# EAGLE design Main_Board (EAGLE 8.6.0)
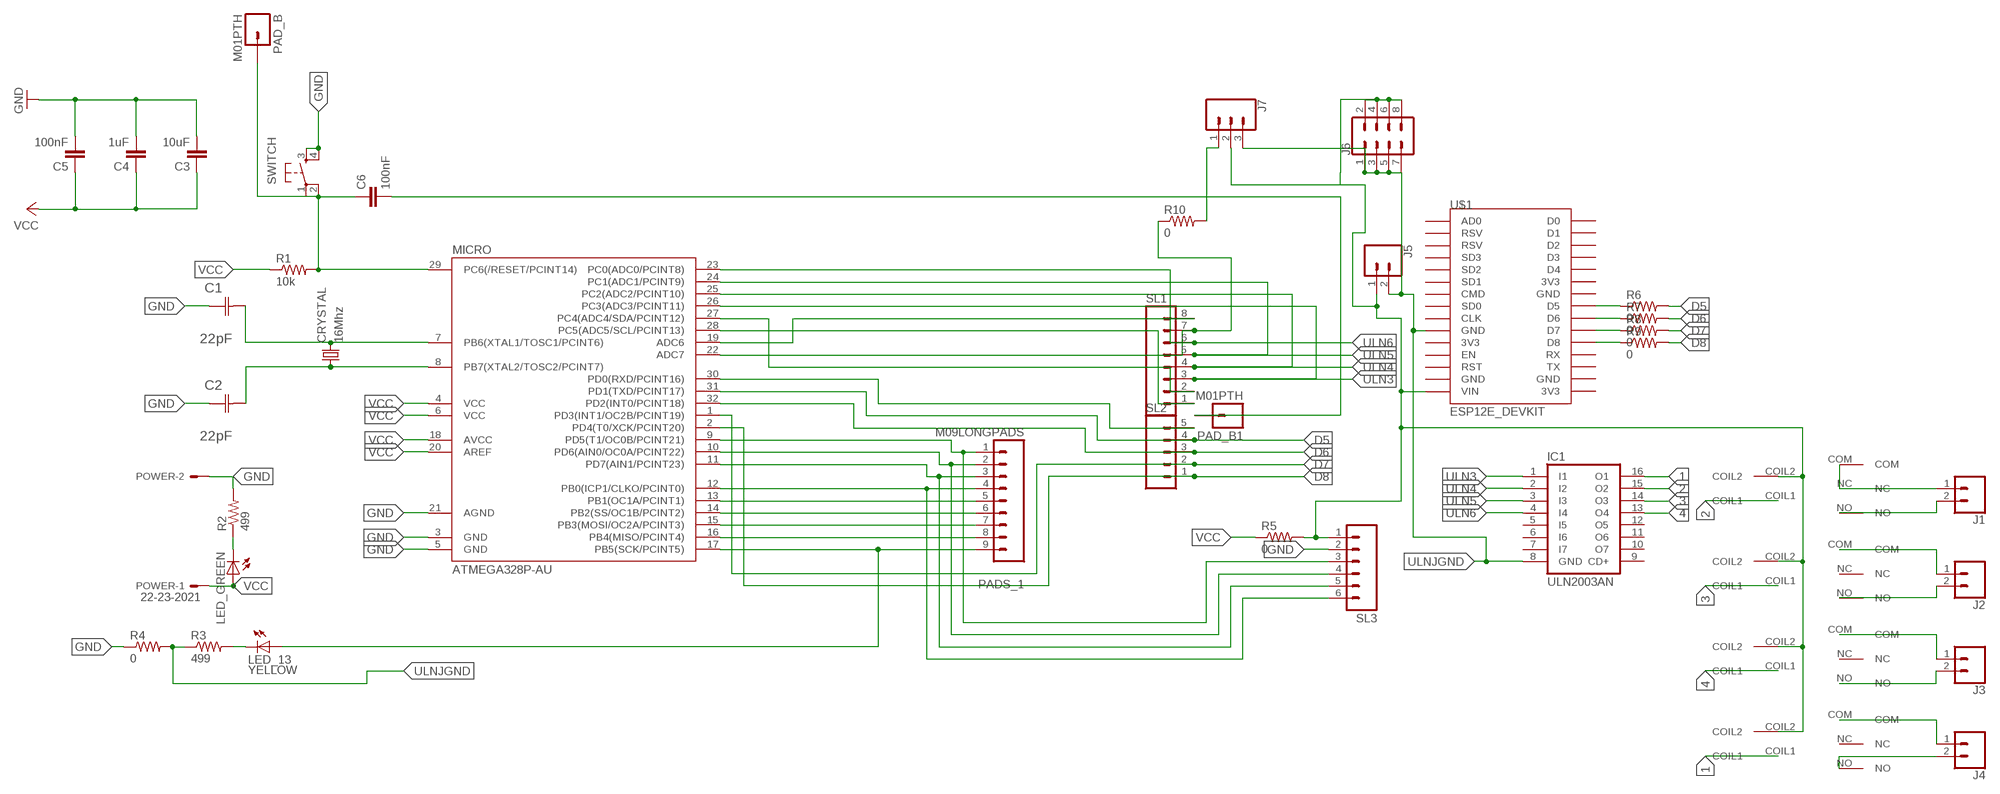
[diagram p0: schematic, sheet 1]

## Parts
C1  22pF  0612ZC225MAT2A  [CAPC3216X178N]
C2  22pF  0612ZC225MAT2A  [CAPC3216X178N]
C3  10uF  CAP1206  [1206]
C4  1uF  CAP1206  [1206]
C5  100nF  CAP1206  [1206]
C6  100nF  CAP1206  [1206]
CRYSTAL  16Mhz  CSM-7X-DU  [CSM-7X-DU]
IC1  ULN2003AN  [DIL16]
J1  CONN_025MM  [SCREWTERMINAL-5MM-2]
J2  CONN_025MM  [SCREWTERMINAL-5MM-2]
J3  CONN_025MM  [SCREWTERMINAL-5MM-2]
J4  CONN_025MM  [SCREWTERMINAL-5MM-2]
J5  CONN_025MM  [SCREWTERMINAL-5MM-2]
J6  CONN_04X2  [2X4]
J7  CONN_03  [1X03]
LED_13  YELLOW  LED1206  [1206]
LED_GREEN  LED1206  [1206]
MICRO  ATMEGA328P-AU  ATMEGA48/88/168-AU  [TQFP32-08]
PAD_B  M01PTH  [1X01]
PAD_B1  M01PTH  [1X01]
PADS_1  M09LONGPADS  [1X09_LONGPADS]
POWER  22-23-2021  [22-23-2021]
R1  10k  RESISTOR1206  [1206]
R2  499  RESISTOR1206  [1206]
R3  499  RESISTOR1206  [1206]
R4  0  RESISTOR1206  [1206]
R5  0  RESISTOR1206  [1206]
R6  0  RESISTOR1206  [1206]
R7  0  RESISTOR1206  [1206]
R8  0  RESISTOR1206  [1206]
R9  0  RESISTOR1206  [1206]
R10  0  RESISTOR1206  [1206]
SL1  M08  [08P]
SL2  M05  [05P]
SL3  M06  [06P]
SWITCH  6MM_SWITCH6MM_SWITCH  [6MM_SWITCH]
U$1  ESP12E_DEVKIT  [ESP12E_DEVKIT]
U$2  1234  [SC05]
U$3  1234  [SC05]
U$4  1234  [SC05]
U$5  1234  [SC05]

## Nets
1: IC1.16(O1) U$5.COIL1
2: IC1.15(O2) U$2.COIL1
3: IC1.14(O3) U$3.COIL1
4: IC1.13(O4) U$4.COIL1
D5: MICRO.31(PD1(TXD/PCINT17)) R6.2 SL2.4
D6: MICRO.32(PD2(INT0/PCINT18)) R7.2 SL2.3
D7: MICRO.1(PD3(INT1/OC2B/PCINT19)) R8.2 SL2.2
D8: MICRO.2(PD4(T0/XCK/PCINT20)) R9.2 SL2.1
GND: C1.1(C1) C2.1(C1) C3.2 C4.2 C5.2 MICRO.3(GND) MICRO.5(GND) MICRO.21(AGND) POWER.2 R2.2 R4.1 SL3.2 SWITCH.3(S) SWITCH.4(S1)
N$1: MICRO.9(PD5(T1/OC0B/PCINT21)) PADS_1.1 SL3.3
N$2: C1.2(C2) CRYSTAL.2 MICRO.7(PB6(XTAL1/TOSC1/PCINT6))
N$3: C6.2 PAD_B1.1
N$4: MICRO.10(PD6(AIN0/OC0A/PCINT22)) PADS_1.2 SL3.4
N$5: MICRO.11(PD7(AIN1/PCINT23)) PADS_1.3 SL3.5
N$6: MICRO.12(PB0(ICP1/CLKO/PCINT0)) PADS_1.4 SL3.6
N$7: MICRO.13(PB1(OC1A/PCINT1)) PADS_1.5
N$8: MICRO.14(PB2(SS/OC1B/PCINT2)) PADS_1.6
N$9: C2.2(C2) CRYSTAL.1 MICRO.8(PB7(XTAL2/TOSC2/PCINT7))
N$10: MICRO.15(PB3(MOSI/OC2A/PCINT3)) PADS_1.7
N$11: MICRO.16(PB4(MISO/PCINT4)) PADS_1.8
N$12: LED_13.1(A) MICRO.17(PB5(SCK/PCINT5)) PADS_1.9
N$13: MICRO.19(ADC6) SL1.8
N$14: MICRO.22(ADC7) R10.1 SL1.7
N$15: J4.2 U$5.NO
N$16: J4.1 U$5.COM
N$17: J7.1 R10.2
N$18: J3.1 U$4.COM
N$19: J3.2 U$4.NO
N$20: MICRO.30(PD0(RXD/PCINT16)) SL2.5
N$21: J2.1 U$3.COM
N$22: J2.2 U$3.NO
N$23: J1.1 U$2.COM
N$24: J1.2 U$2.NO
N$25: J5.1 J6.2 J6.4 J6.6 J6.8 J7.2 R5.2 SL3.1 U$1.VIN U$2.COIL2 U$3.COIL2 U$4.COIL2 U$5.COIL2
N$26: LED_GREEN.2(C) R2.1
N$27: LED_13.2(C) R3.2
N$28: C6.1 MICRO.29(PC6(/RESET/PCINT14)) PAD_B.1 R1.2 SWITCH.1(P) SWITCH.2(P1)
N$31: R9.1 U$1.D8
N$32: R8.1 U$1.D7
N$33: R7.1 U$1.D6
N$34: R6.1 U$1.D5
ULN1: MICRO.28(PC5(ADC5/SCL/PCINT13)) SL1.1
ULN2: MICRO.27(PC4(ADC4/SDA/PCINT12)) SL1.2
ULN3: IC1.1(I1) MICRO.26(PC3(ADC3/PCINT11)) SL1.3
ULN4: IC1.2(I2) MICRO.25(PC2(ADC2/PCINT10)) SL1.4
ULN5: IC1.3(I3) MICRO.24(PC1(ADC1/PCINT9)) SL1.5
ULN6: IC1.4(I4) MICRO.23(PC0(ADC0/PCINT8)) SL1.6
ULNJGND: IC1.8(GND) J5.2 J6.1 J6.3 J6.5 J6.7 J7.3 R3.1 R4.2 U$1.GND@0(GND)
VCC: C3.1 C4.1 C5.1 LED_GREEN.1(A) MICRO.4(VCC) MICRO.6(VCC) MICRO.18(AVCC) MICRO.20(AREF) POWER.1 R1.1 R5.1
Unconnected: IC1.5(I5) IC1.6(I6) IC1.7(I7) IC1.9(CD+) IC1.10(O7) IC1.11(O6) IC1.12(O5) U$1.3V3@0(3V3) U$1.3V3@1(3V3) U$1.3V3@2(3V3) U$1.AD0 U$1.CLK U$1.CMD U$1.D0 U$1.D1 U$1.D2 U$1.D3 U$1.D4 U$1.EN U$1.GND@1(GND) U$1.GND@2(GND) U$1.GND@3(GND) U$1.RST U$1.RSV@0(RSV) U$1.RSV@1(RSV) U$1.RX U$1.SD0 U$1.SD1 U$1.SD2 U$1.SD3 U$1.TX U$2.NC U$3.NC U$4.NC U$5.NC

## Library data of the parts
C1 C2 = AVX_By_element14_Batch_1:0612ZC225MAT2A: Capacitor 1206; MPN: 0612ZC225MAT2A; OC_FARNELL: -; OC_NEWARK: 12N3209; SUPPLIER: AVX; TOLERANCE: ±20%; VALUE: 2.2µF; VOLTAGERATING: 10V
C3-C6 = 01_SparkFun:CAP: Capacitor
CRYSTAL = 01_FAB_Hello:CSM-7X-DU: SMD CRYSTAL; OC_FARNELL: unknown; OC_NEWARK: unknown
IC1 = uln-udn:ULN2003A: DRIVER ARRAY
J1-J5 = SparkFun-Connectors:CONN_02: Multi connection point. Often used as Generic Header-pin footprint for 0.1 inch spaced/style header connections; SF_SKU: PRT-08432
J6 = SparkFun-Connectors:CONN_04X2: Multi connection point. Often used as Generic Header-pin footprint for 0.1 inch spaced/style header connections On any of the 0.1 inch spaced packages, you can populate with these: Break Away Headers - Straight (PRT-00116) Break Away Male Headers - Right Angle (PRT-00553) Female Headers (PRT-00115)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
J7 = SparkFun-Connectors:CONN_03: Multi connection point. Often used as Generic Header-pin footprint for 0.1 inch spaced/style header connections On any of the 0.1 inch spaced packages, you can populate with these: Break Away Headers - Straight (PRT-00116) Break Away Male Headers - Right Angle (PRT-00553) Female Headers (PRT-00115)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
LED_13 LED_GREEN = 01_FAB_Hello:LED
MICRO = atmega8:ATMEGA48/88/168
PAD_B PAD_B1 = 01_SparkFun:M01: Header 1
PADS_1 = 01_SparkFun:M09: Header 9 Standard 9-pin 0.1" header. Use with straight break away headers (SKU : PRT-00116), right angle break away headers (PRT-00553), swiss pins (PRT-00743), machine pins (PRT-00117), and female headers (PRT-00115).
POWER = con-molex:22-23-2021: .100" (2.54mm) Center Header - 2 Pin; MF: MOLEX; MPN: 22-23-2021; OC_FARNELL: 1462926; OC_NEWARK: 25C3832
R1-R10 = 01_SparkFun:RESISTOR: Resistor
SL1 = con-amp-quick:M08: AMP QUICK CONNECTOR; OC_FARNELL: unknown; OC_NEWARK: unknown
SL2 = con-amp-quick:M05: AMP QUICK CONNECTOR; OC_FARNELL: unknown; OC_NEWARK: unknown
SL3 = con-amp-quick:M06: AMP QUICK CONNECTOR; OC_FARNELL: unknown; OC_NEWARK: unknown
SWITCH = 01_FAB_Hello:6MM_SWITCH: OMRON SWITCH
U$1 = nodemcu:ESP12E_DEVKIT: ESP12E DEVKIT BOARD
U$2-U$5 = realySC05:1234

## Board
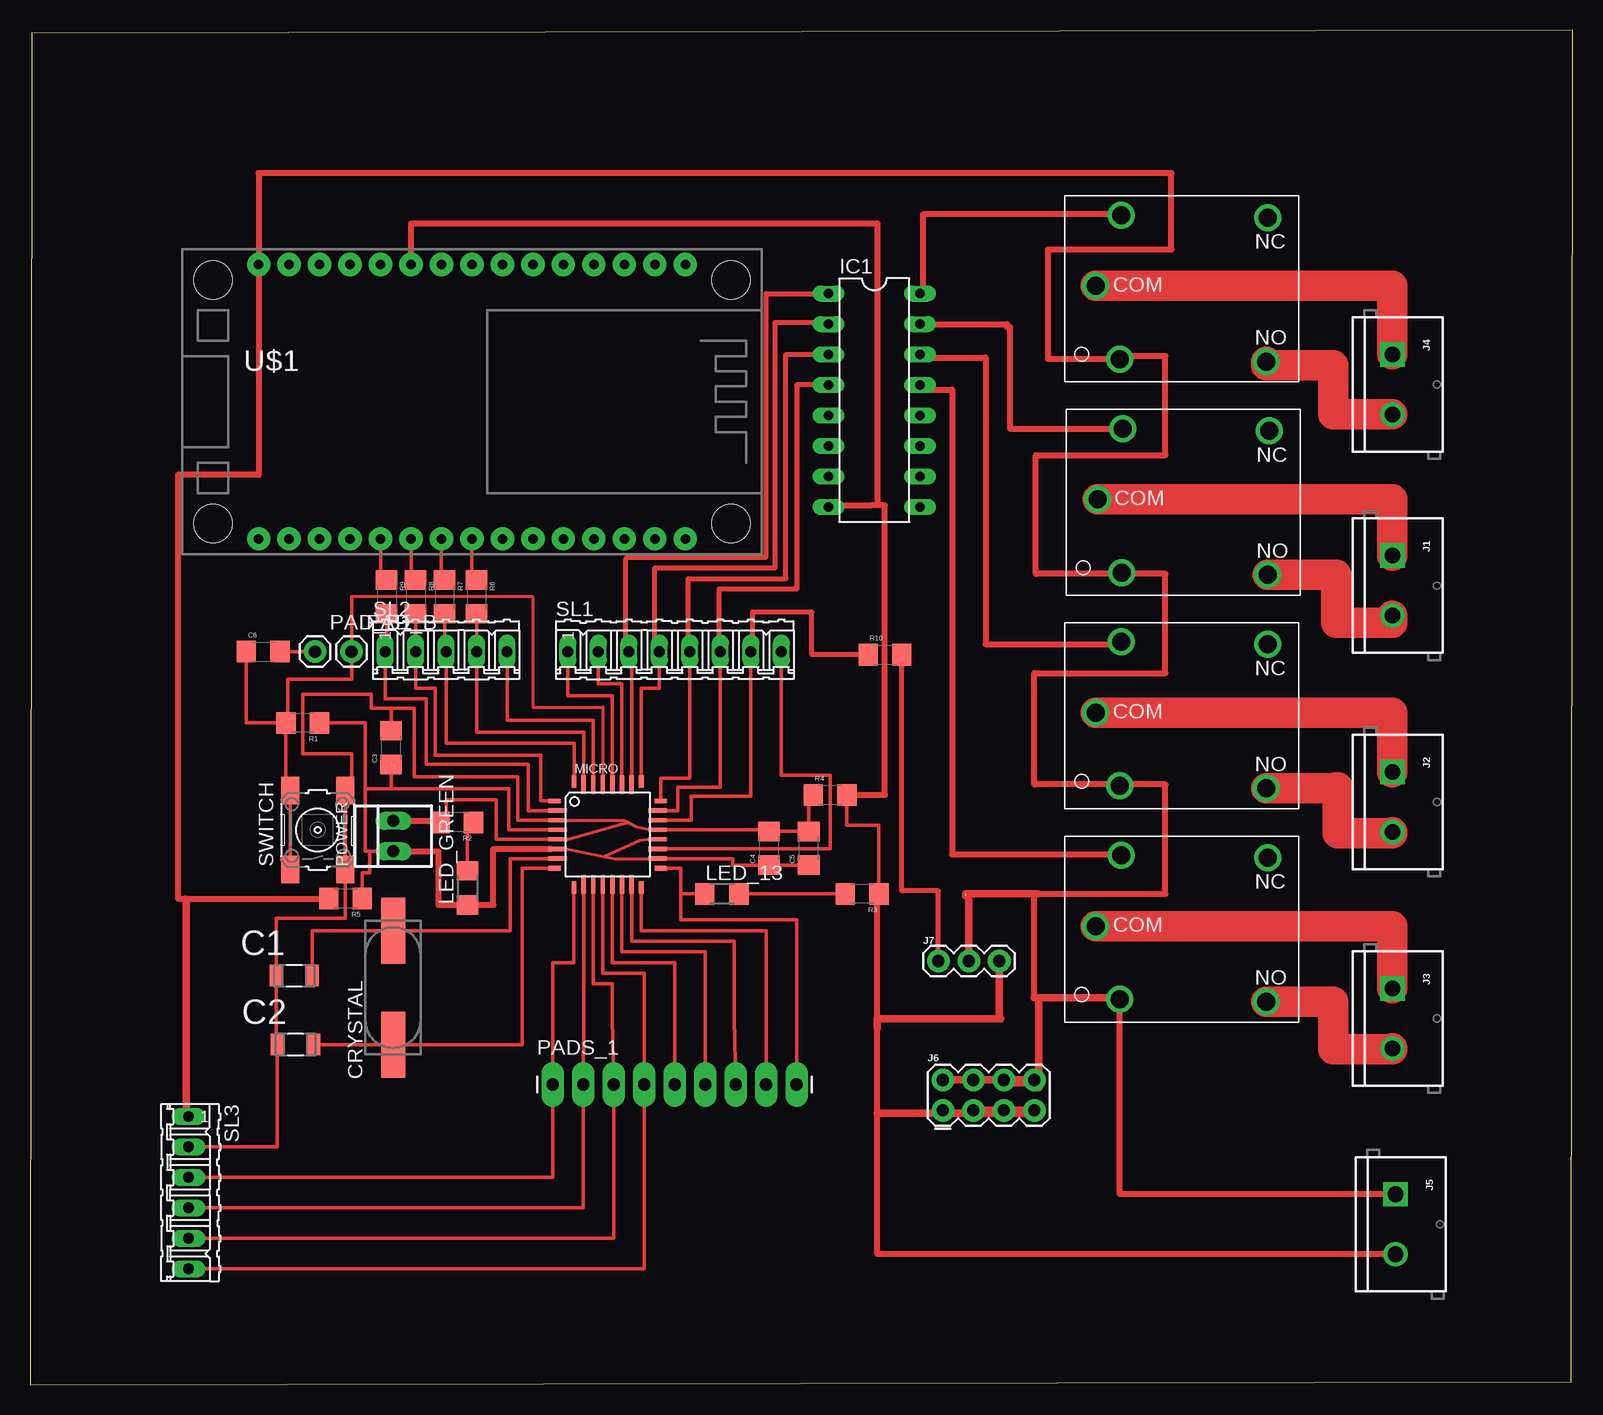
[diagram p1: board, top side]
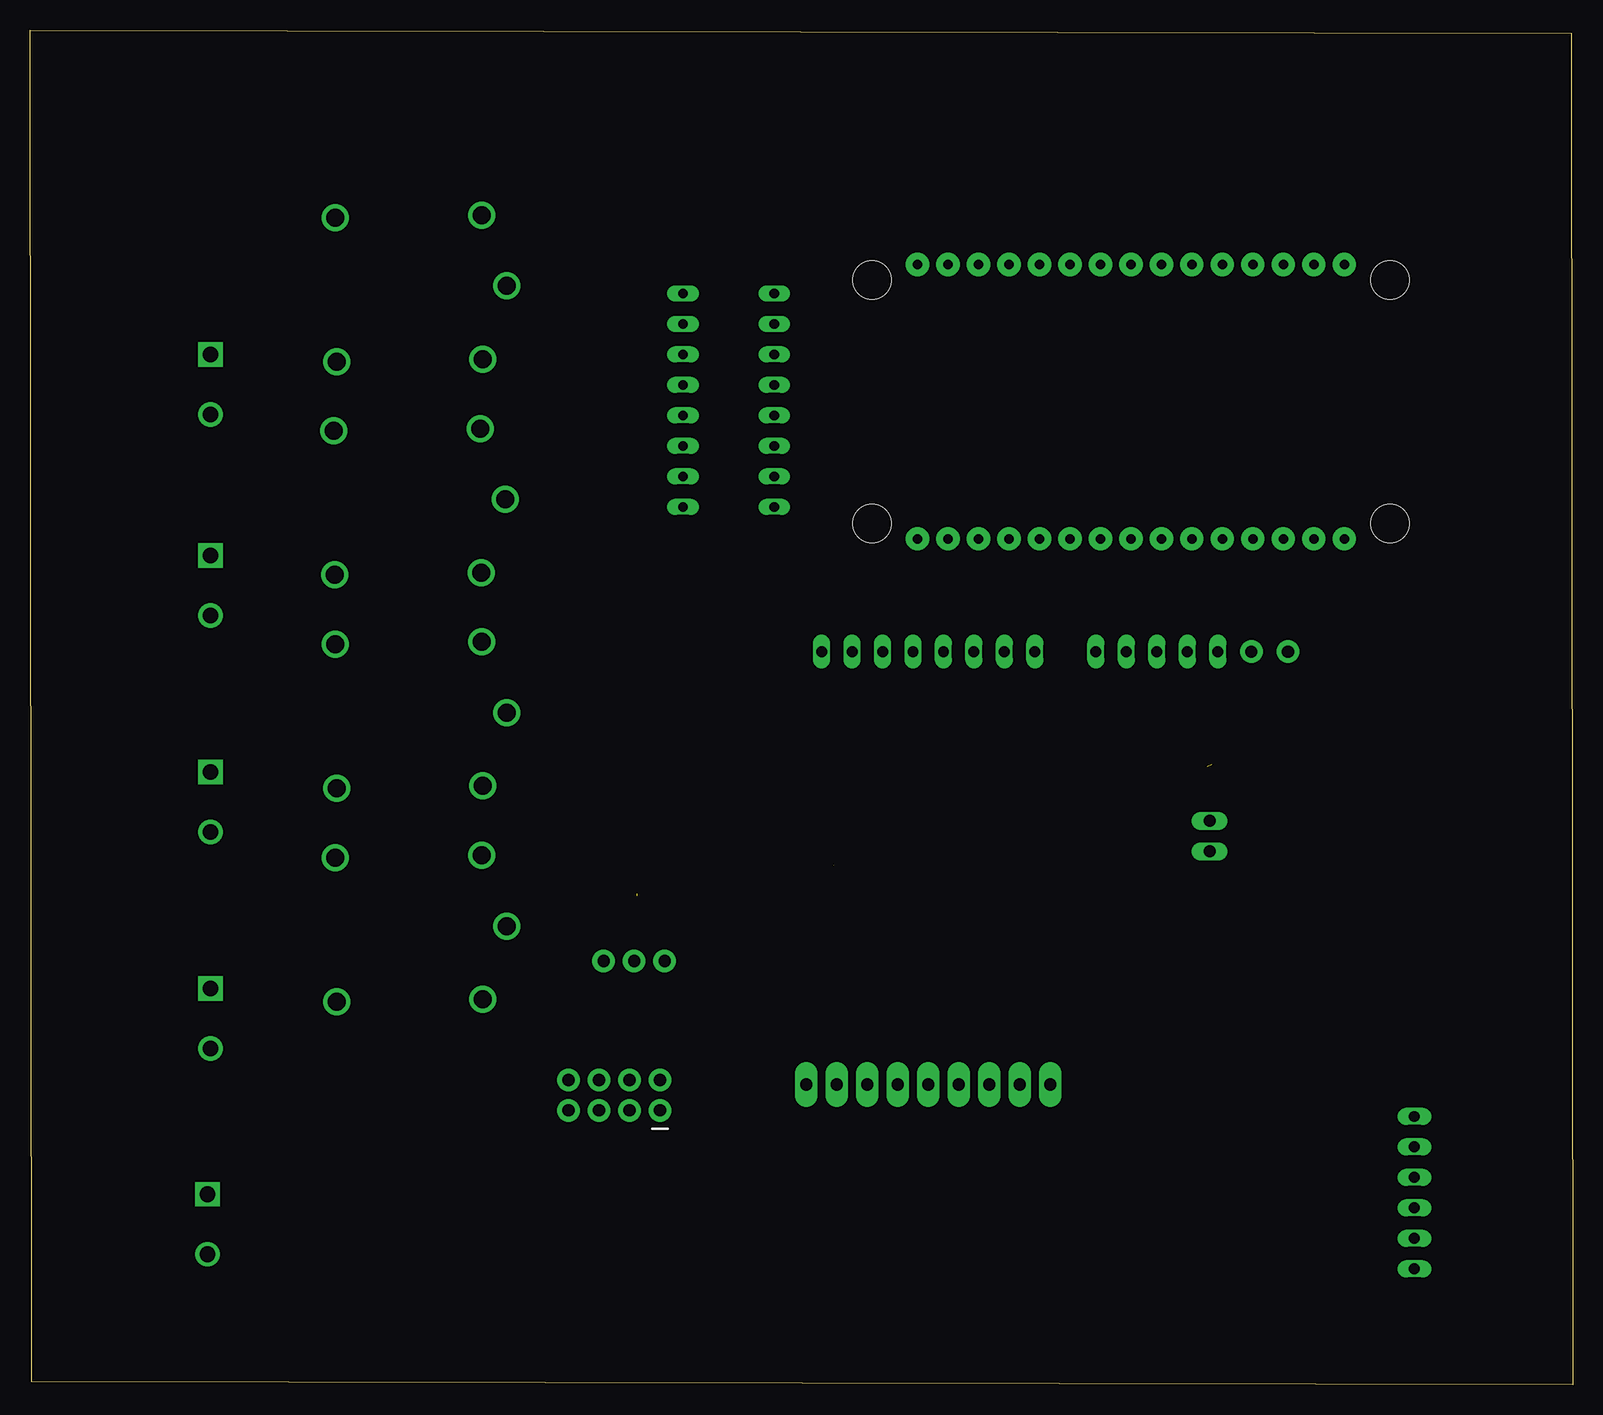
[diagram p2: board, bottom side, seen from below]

Size 128.57 x 112.89 mm. Coordinates in mm from the lower left corner, seen from the top.
Outline: 0,0 128.45,0.25 128.57,112.89 0.13,112.64 0,0
Copper layers (1*16): Top 0.035mm / dielectric 1.5mm / Bottom 0.035mm
Design rules "default": minimum track width 10mil, minimum drill 24mil, track to track 8mil, track to pad 8mil, pad to pad 8mil, via to via 8mil, smd to smd 8mil, copper to edge 40mil, drill to drill 8mil, minimum pad ring 10mil, minimum via ring 8mil, stop-mask expansion 4mil, vias tented up to drill 0mil, thermal gap 10mil

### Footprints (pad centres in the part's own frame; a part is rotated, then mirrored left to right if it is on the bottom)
CAPC3216X178N = smd 1.118 x 1.803: 1 -1.499,0; 2 1.499,0
1206 = smd 1.6 x 1.8: 1 -1.4,0; 2 1.4,0
CSM-7X-DU = smd 5.5 x 2: 1 -4.75,0; 2 4.75,0
DIL16 = drill 0.813 long: 1 -8.89,-3.81; 2 -6.35,-3.81; 3 -3.81,-3.81; 4 -1.27,-3.81; 5 1.27,-3.81; 6 3.81,-3.81; 7 6.35,-3.81; 8 8.89,-3.81; 9 8.89,3.81; 10 6.35,3.81; 11 3.81,3.81; 12 1.27,3.81; 13 -1.27,3.81; 14 -3.81,3.81; 15 -6.35,3.81; 16 -8.89,3.81
SCREWTERMINAL-5MM-2 = drill 1.3 pad 2.032 square: 1 0,0 | drill 1.3 pad 2.032: 2 5,0
2X4 = drill 1.016 pad 1.88: 1 -3.81,-1.27; 2 -3.81,1.27; 3 -1.27,-1.27; 4 -1.27,1.27; 5 1.27,-1.27; 6 1.27,1.27; 7 3.81,-1.27; 8 3.81,1.27
1X03 = drill 1.016 pad 1.88: 1 0,0; 2 2.54,0; 3 5.08,0
1206' = smd 1.6 x 1.803: 1 -1.422,0; 2 1.422,0
TQFP32-08 = smd 1.016 x 0.406: 1 -4.42,2.8; 8 -4.42,-2.8; 17 4.42,-2.8; 24 4.42,2.8 | smd 1.524 x 0.356: 2 -4.166,2; 3 -4.166,1.2; 4 -4.166,0.4; 5 -4.166,-0.4; 6 -4.166,-1.2; 7 -4.166,-2; 18 4.166,-2; 19 4.166,-1.2; 20 4.166,-0.4; 21 4.166,0.4; 22 4.166,1.2; 23 4.166,2 | smd 0.406 x 1.016: 9 -2.8,-4.42; 16 2.8,-4.42; 25 2.8,4.42; 32 -2.8,4.42 | smd 0.356 x 1.524: 10 -2,-4.166; 11 -1.2,-4.166; 12 -0.4,-4.166; 13 0.4,-4.166; 14 1.2,-4.166; 15 2,-4.166; 26 2,4.166; 27 1.2,4.166; 28 0.4,4.166; 29 -0.4,4.166; 30 -1.2,4.166; 31 -2,4.166
1X01 = drill 1.016 pad 1.88: 1 0,0
1X09_LONGPADS = drill 1.016 pad 1.88 long: 1 0,0; 2 2.54,0; 3 5.08,0; 4 7.62,0; 5 10.16,0; 6 12.7,0; 7 15.24,0; 8 17.78,0; 9 20.32,0
22-23-2021 = drill 1 long: 1 -1.27,0; 2 1.27,0
08P = drill 0.914 long: 1 -8.89,0; 2 -6.35,0; 3 -3.81,0; 4 -1.27,0; 5 1.27,0; 6 3.81,0; 7 6.35,0; 8 8.89,0
05P = drill 0.914 long: 1 -5.08,0; 2 -2.54,0; 3 0,0; 4 2.54,0; 5 5.08,0
06P = drill 0.914 long: 1 -6.35,0; 2 -3.81,0; 3 -1.27,0; 4 1.27,0; 5 3.81,0; 6 6.35,0
6MM_SWITCH = smd 2.286 x 1.524: 1 -3.302,2.286; 2 3.302,2.286; 3 -3.302,-2.286; 4 3.302,-2.286
ESP12E_DEVKIT = drill 0.8 pad 1.93: 3V3@0 -11.43,-7.62; 3V3@1 11.43,5.08; 3V3@2 11.43,-17.78; AD0 -11.43,17.78; CLK -11.43,-2.54; CMD -11.43,2.54; D0 11.43,17.78; D1 11.43,15.24; D2 11.43,12.7; D3 11.43,10.16; D4 11.43,7.62; D5 11.43,0; D6 11.43,-2.54; D7 11.43,-5.08; D8 11.43,-7.62; EN -11.43,-10.16; GND@0 -11.43,-5.08; GND@1 -11.43,-15.24; GND@2 11.43,2.54; GND@3 11.43,-15.24; RST -11.43,-12.7; RSV@0 -11.43,15.24; RSV@1 -11.43,12.7; RX 11.43,-10.16; SD0 -11.43,0; SD1 -11.43,5.08; SD2 -11.43,7.62; SD3 -11.43,10.16; TX 11.43,-12.7; VIN -11.43,-17.78 | hole 3.2: -10.16,21.59; 10.16,21.59; 10.16,-21.59; -10.16,-21.59
SC05 = drill 1.5: COIL1 4.7,-1.6; COIL2 4.6,-13.6; COM 2.6,-7.5; NC 16.9,-1.8; NO 16.8,-13.8

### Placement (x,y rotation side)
C1  22.02,34.09 0 top
C2  22.12,28.35 0 top
C3  30.1,53.09 90 top
C4  61.59,44.7 90 top
C5  64.9,44.7 90 top
C6  19.43,61.09 0 top
CRYSTAL  30.25,33.1 90 top
IC1  70.36,82.04 270 top
J1  113.54,69.09 270 top
J2  113.54,51.05 270 top
J3  113.54,33.02 270 top
J4  113.54,85.85 270 top
J5  113.79,15.88 270 top
J6  79.88,24.13 0 top
J7  75.69,35.31 0 top
LED_13  YELLOW  [1206']  57.66,40.89 0 top
LED_GREEN  [1206']  36.45,41.4 90 top
MICRO  48.13,45.85 0 top
PAD_B  26.8,61.09 0 top
PAD_B1  23.75,61.09 0 top
PADS_1  43.56,25.02 0 top
POWER  30.28,45.72 90 top
R1  22.73,55.14 180 top
R2  35.56,46.86 180 top
R3  69.34,40.89 180 top
R4  66.67,49.15 0 top
R5  26.29,40.51 180 top
R6  37.21,65.66 270 top
R7  34.54,65.66 270 top
R8  32.13,65.66 270 top
R9  29.72,65.66 270 top
R10  71.25,60.83 0 top
SL1  53.72,61.09 0 top
SL2  34.67,61.09 0 top
SL3  13.21,16 270 top
SWITCH  23.98,46.23 90 top
U$1  36.83,81.92 270 top
U$2  86.36,81.28 0 top
U$3  86.23,63.5 0 top
U$4  86.23,45.72 0 top
U$5  86.23,99.06 0 top

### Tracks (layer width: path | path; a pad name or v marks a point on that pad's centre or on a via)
1
  Top 0.508: IC1.16 74.42,90.93 74.42,97.54 90.93,97.54 U$5.COIL1
2
  Top 0.305: 81.66,79.68 U$2.COIL1
  Top 0.508: IC1.15 81.41,88.39 81.41,88.14 81.66,88.14 81.66,79.68 91.57,79.68 91.57,79.38 91.06,79.38 U$2.COIL1
3
  Top 0.305: 91.31,61.72 91.31,61.47
  Top 0.508: U$3.COIL1 90.93,61.72 | 90.93,61.72 91.31,61.72 | IC1.14 74.17,85.6 79.63,85.6 79.63,61.72 90.93,61.72
4
  Top 0.305: U$4.COIL1 90.93,44.2 90.55,44.2
  Top 0.508: IC1.13 74.17,82.93 76.84,82.93 76.84,44.2 90.55,44.2
D5
  Top 0.305: MICRO.31 46.13,54.36 37.21,54.36 37.21,60.33 SL2.4 R6.2
D6
  Top 0.305: MICRO.32 45.34,53.47 34.67,53.47 34.67,60.71 | SL2.3 34.67,60.71 | R7.2 34.54,60.71 34.67,60.71
D7
  Top 0.305: MICRO.1 42.55,48.65 42.55,52.45 33.78,52.45 33.78,58.04 32.13,58.04 32.13,60.45 SL2.2 R8.2
D8
  Top 0.305: MICRO.2 41.53,47.85 41.53,51.69 33.02,51.69 33.02,57.15 29.59,57.15 29.59,60.71 | 29.59,60.71 SL2.1 29.72,61.09 R9.2 29.72,60.71 29.59,60.71
GND
  Top 0.254: MICRO.3 43.99,47.02 49.52,47.02 | 49.52,47.02 50.55,46.48 51.69,46.23 | 44.58,45.47 44.83,45.47 49.71,46.81 | 49.71,46.81 49.84,46.85 | 49.52,47.02 49.71,46.81
  Top 0.305: MICRO.5 | MICRO.21 | 20.52,28.35 C2.1 20.62,27.81 | MICRO.5 43.97,45.47 38.86,45.47 38.86,48.77 34.67,48.77 34.67,46.74 R2.2 34.67,46.99 | MICRO.21 61.59,46.25 C4.2 C5.2 64.9,49.15 R4.1 | 44.58,45.47 MICRO.5 | MICRO.21 51.69,46.23 | MICRO.3 40.64,47.05 40.64,50.67 32,50.67 32,56.39 30.1,56.39 | 30.1,56.39 28.45,56.39 28.45,57.53 22.73,57.53 22.73,52.58 26.8,52.58 26.8,49.4 SWITCH.4 SWITCH.3 26.26,38.86 20.52,38.86 C1.1 20.52,27.81 20.62,27.81 | C3.2 30.1,56.39 | 20.62,27.81 20.62,19.81 SL3.2
  Top 0.508: POWER.2 34.67,46.99
N$1
  Top 0.305: MICRO.9 45.33,35.18 43.56,35.18 PADS_1.1 43.56,17.27 SL3.3
N$2
  Top 0.305: 23.52,37.85 C1.2 23.52,37.85 | MICRO.7 43.97,43.82 40.01,43.82 40.01,37.85 CRYSTAL.2 23.52,37.85
N$3
  Top 0.305: PAD_B1.1 C6.2
N$4
  Top 0.305: MICRO.10 46.13,30.48 PADS_1.2 46.1,14.73 SL3.4
N$5
  Top 0.305: MICRO.11 46.93,33.4 48.51,33.4 48.51,30.48 PADS_1.3 48.64,12.19 SL3.5
N$6
  Top 0.305: 47.75,41.68 MICRO.12 47.73,34.29 51.18,34.29 PADS_1.4 51.18,9.65 SL3.6
N$7
  Top 0.305: PADS_1.5 53.72,35.18 48.53,35.18 MICRO.13
N$8
  Top 0.305: PADS_1.6 56.26,36.07 49.33,36.07 MICRO.14
N$9
  Top 0.305: 23.62,28.32 C2.2 | MICRO.8 41.02,43.05 41.02,28.35 CRYSTAL.1 C2.2 | C2.2
N$10
  Top 0.305: PADS_1.7 58.67,30.48 58.67,36.96 50.16,36.96 50.16,40.89 MICRO.15
N$11
  Top 0.305: MICRO.16 50.93,37.85 61.34,37.85 PADS_1.8
N$12
  Top 0.305: PADS_1.9 63.88,38.73 54.23,38.73 54.23,40.89 | LED_13.1 54.23,40.89 | MICRO.17 54.23,43.05 54.23,40.89
N$13
  Top 0.305: MICRO.19 66.67,44.65 66.67,50.8 62.61,50.8 SL1.8
N$14
  Top 0.305: MICRO.22 55.12,47.05 55.12,49.02 60.07,49.02 SL1.7
  Top 0.406: R10.1 65.15,60.83 65.15,64.39 60.2,64.39 60.2,61.09 SL1.7
N$15
  Top 2.54: U$5.NO 103.03,84.96 108.59,84.96 108.59,80.85 J4.2
N$16
  Top 2.54: U$5.COM 113.54,91.56 J4.1
N$17
  Top 0.406: J7.1 75.69,41.15 72.65,41.15 R10.2
N$18
  Top 2.54: U$4.COM 113.54,38.22 J3.1
N$19
  Top 2.54: U$4.NO 108.59,31.92 108.59,27.94 113.54,27.94 J3.2
N$20
  Top 0.305: MICRO.30 46.93,55.37 39.75,55.37 SL2.5
N$21
  Top 2.54: U$3.COM 113.54,56 J2.1
N$22
  Top 2.54: U$3.NO 108.84,49.7 108.84,49.78 108.97,49.78 108.97,45.97 113.54,45.97 J2.2
N$23
  Top 2.54: U$2.COM 113.54,73.78 J1.1
N$24
  Top 2.54: U$2.NO 108.84,67.48 108.84,63.5 113.54,63.5 J1.2
N$25  (1 unrouted)
  Top 0.305: SL3.1 13.21,22.61 13.21,40.51 | 13.21,40.51 24.38,40.51 R5.2 | U$1.VIN 19.05,92.84 19.05,75.82 | 12.95,40.51 13.21,40.51
  Top 0.508: 90.83,32.26 84.07,32.26 83.69,32.26 83.69,40.89 83.95,40.89 94.62,40.89 94.62,50.04 91.06,50.04 | 90.96,67.56 94.62,67.56 94.62,59.31 83.69,59.31 83.69,50.04 91.06,50.04 | 90.96,67.56 83.82,67.56 83.82,77.47 94.62,77.47 94.62,85.72 90.83,85.72 U$5.COIL2 84.84,85.46 84.84,94.62 95.12,94.62 95.12,100.97 19.05,100.97 19.05,92.84 | U$2.COIL2 90.96,67.56 | U$3.COIL2 91.06,49.9 91.06,50.04 | U$1.VIN 19.05,75.82 12.32,75.82 12.32,40.51 12.95,40.51 | 12.95,40.51 24.38,40.51 | 12.95,40.51 12.95,22.61 13.21,22.61 | J5.1 90.83,15.88 U$4.COIL2
  Top 0.61: 84.07,32.26 84.07,25.15 | 84.07,25.15 84.07,24.77 83.69,24.77 J6.8 J6.4 J6.2 | J6.6 81.15,25.15 84.07,25.15 | U$4.COIL2 90.83,32.26 83.69,32.26 | J7.2 78.23,40.77 77.98,40.77 | 77.98,40.89 83.95,40.89
N$26
  Top 0.305: 37.34,46.61 R2.1 36.96,46.48 36.45,46.48 LED_GREEN.2
N$27
  Top 0.305: LED_13.2 R3.2
N$28
  Top 0.254: 26.8,65.66 41.91,65.66 41.91,56.46 47.73,56.46 MICRO.29
  Top 0.305: SWITCH.1 SWITCH.2 | SWITCH.2 22.09,49.53 | SWITCH.2 21.33,49.53 R1.2 | R1.2 21.08,55.14 | C6.1 18.03,55.14 R1.2 | R1.2 21.46,55.14 21.46,58.8 26.8,58.8 26.8,60.83 | 26.8,60.83 PAD_B.1 26.8,65.66 | 26.92,60.83 26.8,60.83
  Top 0.406: SWITCH.1 21.59,42.93
N$31
  Top 0.305: U$1.D8 29.21,67.06 R9.1
N$32
  Top 0.305: U$1.D7 31.75,67.06 R8.1
N$33
  Top 0.305: U$1.D6 34.29,67.06 R7.1
N$34
  Top 0.305: U$1.D5 36.83,67.06 R6.1
ULN1
  Top 0.305: MICRO.28 48.51,50.01 48.51,57.4 44.83,57.4 SL1.1
ULN2
  Top 0.305: MICRO.27 49.33,58.42 47.37,58.42 SL1.2
ULN3
  Top 0.305: MICRO.26 50.16,50.01 50.16,61.09 SL1.3
  Top 0.406: SL1.3 49.66,61.09 49.66,68.83 49.76,68.94 59.59,68.94 59.61,68.96 61.34,68.96 61.34,90.93 IC1.1
ULN4
  Top 0.305: MICRO.25 50.93,58.04 52.45,58.04 SL1.4
  Top 0.406: SL1.4 52.07,61.09 52.07,68.07 62.1,68.07 62.1,88.52 66.55,88.52 IC1.2
ULN5
  Top 0.305: MICRO.24 52.58,48.65 52.58,50.55 54.99,50.55 SL1.5
  Top 0.406: SL1.5 54.86,61.09 54.86,67.18 62.99,67.18 62.99,85.85 IC1.3
ULN6
  Top 0.305: MICRO.23 53.98,47.85 53.98,49.78 57.53,49.78 57.53,60.71 SL1.6
  Top 0.406: IC1.4 63.88,83.31 63.88,66.29 57.4,66.29 57.4,60.71 57.53,60.71
ULNJGND
  Top 0.305: R3.1 70.74,46.61 68.08,46.61 R4.2 | 70.1,73.28 70.61,73.28 70.61,73.66
  Top 0.508: R4.2 71.25,49.15 71.25,73.28 70.1,73.28 66.55,73.28 IC1.8 | U$1.GND@0 31.75,96.77 70.61,96.77 70.61,73.66 | J5.2 70.61,10.88 70.61,22.61 70.61,29.72 70.61,40.89 R3.1
  Top 0.61: J6.1 76.07,22.61 78.61,22.61 | 79.38,22.61 78.61,22.61 | 78.61,22.61 J6.3 J6.5 J6.7 83.69,22.61 70.61,22.61 | J7.3 80.77,30.48 | 80.77,30.48 80.9,30.48 | 80.77,30.48 70.61,30.48 70.61,29.72
VCC  (2 unrouted)
  Top 0.254: 44.65,44.65 47.11,44.15 47.87,44 | 47.87,44 48.77,43.82 52.3,43.82 | MICRO.20 51.69,45.45 51.69,45.47 50.8,45.34 47.87,44
  Top 0.305: MICRO.18 | MICRO.20 51.69,45.47 | MICRO.4 39.88,46.25 39.88,49.66 30.1,49.66 | 27.94,49.66 27.94,55.14 R1.1 | 27.94,49.66 27.94,44.45 28.32,44.45 | POWER.1 28.32,44.45 | 52.3,43.82 MICRO.18 | 34.04,44.45 34.04,44.2 | 43.43,44.65 MICRO.6 44.65,44.65 | MICRO.18 58.55,43.85 58.55,43.31 C4.1 | 30.48,51.56 30.48,51.44 | 27.94,49.66 30.1,49.66 | 30.1,49.66 C3.1 | C4.1 C5.1 | R5.1 27.69,42.67 28.32,42.67 28.32,44.45
  Top 0.508: POWER.1 34.04,44.45 | 34.04,44.2 34.04,39.98 LED_GREEN.1 38.61,39.98 38.61,44.65 43.43,44.65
